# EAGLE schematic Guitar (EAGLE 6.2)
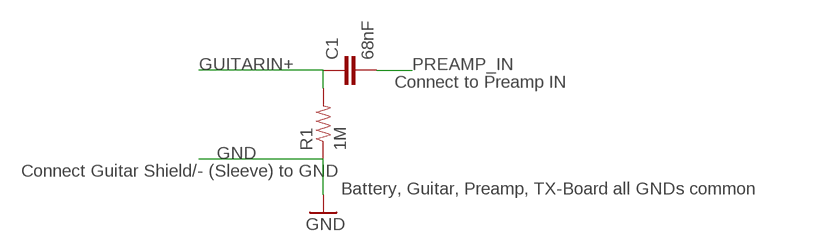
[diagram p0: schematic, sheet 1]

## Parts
C1  68nF  CAPPTH  [CAP-PTH-SMALL]
R1  1M  RESISTORAXIAL-0.3  [AXIAL-0.3]

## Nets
GND: R1.P$1
GUITARIN+: C1.1 R1.P$2
PREAMP_IN: C1.2

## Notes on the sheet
- Connect to Preamp IN
- Connect Guitar Shield/- (Sleeve) to GND
- Battery, Guitar, Preamp, TX-Board all GNDs common

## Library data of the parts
C1 = SparkFun-Passives:CAP: Capacitor
R1 = SparkFun-Passives:RESISTOR: Resistor

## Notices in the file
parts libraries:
SparkFun-Passives: Licensing: CC v3.0 Share-Alike You are welcome to use this library for commercial purposes.
